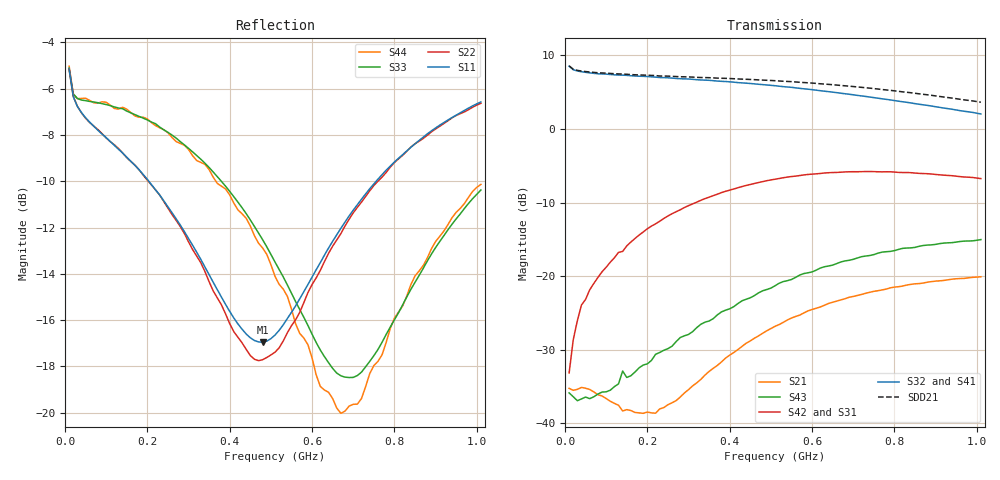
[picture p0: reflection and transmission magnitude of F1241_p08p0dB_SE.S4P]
! Integrated Device Technology
! Corporate Headquarters
! 6024 Silver Creek Valley Road
! San Jose, CA 95138  USA
! Phone:  1-408-284-8200
! Toll Free:  1-800-223-1366
! Webpage:  http://www.idt.com/
! Timing and RF Division
! 515 Groton Road, Suite 102
! Westford, MA 01886-6024
! Device:  F1241
! Description: Dual Intermediate Frequency Digital Variable Gain Amplifier
! Frequency:  10.0 -  500.00 MHz
! Package:  5x5 mm QFN Plastic Package: 32 pin
! Ports:  8 RF, 20 DC
!  Pin  1  = GA3  Pin 17  = RF OUT_B+
!  Pin  2  = GA4  Pin 18  = RF OUT_B-
!  Pin  3  = GA5  Pin 19  = STBY_B
!  Pin  4  = ISET_A  Pin 20  = Ground
!  Pin  5  = ISET_B  Pin 21  = Ground
!  Pin  6  = GB5  Pin 22  = STB_A
!  Pin  7  = GB4  Pin 23  = RF OUT_A-  = Port 4
!  Pin  8  = GB3  Pin 24  = RF OUT_A+  = Port 3
!  Pin  9  = GB2  Pin 25  = NO CONNECT
!  Pin 10  = GB1  Pin 26  = NO CONNECT
!  Pin 11  = RF IN_B+  Pin 27  = VCC
!  Pin 12  = RF IN_B-  Pin 28  = Ground
!  Pin 13  = Ground  Pin 29  = RF IN_A-  = Port 2
!  Pin 14  = VCC  Pin 30  = RF IN_A+  = Port 1
!  Pin 15  = NO CONNECT  Pin 31  = GA1
!  Pin 16  = NO CONNECT  Pin 32  = GA2
!  Pin 16  = GB0  Pin 32  = GA2 / CSb
! State:  12
! Gain State:  8.0 dB
! Voltages:  Vcc = +5.00 Volts  Icc approximately 160.0 mA or 80 mA per channel.
! Data:  The device was measured on a custom evaluation board which has
!  individual transmission lines to the RF pins.  Data was collected
!  using a calibrated network analyzer.  The evaluation board was
!  de-embedded using a port reference technique.
!  The reference plane is the edge of the package pin.
!  Only Channel A was measured.
!  This data is in single-ended operation.  If your needs are balanced
!  or differential S-parameters then this file needs to be used a
!  linear simulator.
! Misc:  Lot Code  160028MY
!  Action Tracker AT004
! Date Measured:  2014-08-14
! Date:  2014-08-28  MJV
! Note:
!  Integrated Device Technology supplies this data as a sample of measured
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# Hz S dB R 50
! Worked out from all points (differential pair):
!   101 points, 10 MHz to 1.01 GHz, reference 50 ohm
!   strongest paths, dB at 10 MHz, 260 MHz, 510 MHz, 760 MHz, 1.01 GHz:
!     S32: 8.5, 6.9, 5.9, 4.2, 2.0
!     S41: 8.6, 6.9, 5.8, 4.1, 1.9
!     S42: -33.2, -11.5, -6.8, -5.8, -6.7
!     S31: -33.1, -11.5, -6.9, -5.9, -6.8
!     S43: -35.9, -29.5, -21.3, -16.9, -15.0
!     S21: -35.2, -37.2, -26.8, -22.0, -20.1
!   taken as a pair (ports 2,1 in; 3,4 out), SDD21 dB: 8.6, 7.2, 6.6, 5.4, 3.6
!   lowest |S11| = -17.0 dB at 480 MHz (marker M1), VSWR 1.33, Z = 39.9 - j7.86 ohm
!   |S11| at or under -10 dB: 203.7 MHz to 755.6 MHz (551.9 MHz wide, 115 % of centre)
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1e7  -5.15 -22.0  -35.26 -9.2  -60.41 64.0  -17.31 14.8
     -35.25 -9.6  -5.17 -21.7  -17.34 14.5  -59.31 65.2
     -33.12 64.3  8.53 177.8  -5.11 -20.5  -36.02 176.5
     8.56 177.9  -33.16 63.4  -35.87 176.6  -5.03 -20.6
5e7  -7.25 -18.7  -35.29 -1.8  -45.83 74.4  -17.35 -1.6
     -35.24 -1.9  -7.28 -18.2  -17.31 -1.7  -45.95 75.4
     -23.06 58.0  7.70 170.0  -6.52 -9.4  -36.66 158.6
     7.71 169.7  -23.16 57.7  -36.43 156.4  -6.41 -9.4
1.4e8  -8.78 -32.0  -38.07 11.6  -37.58 68.9  -17.58 -8.3
       -38.33 8.6  -8.78 -30.6  -17.53 -8.1  -37.58 68.8
       -16.60 52.9  7.31 157.4  -6.87 -16.1  -33.44 145.0
       7.31 156.9  -16.64 52.5  -32.90 142.4  -6.80 -15.3
3.2e8  -13.07 -69.0  -33.44 67.5  -31.21 51.4  -17.26 -17.3
       -34.50 69.0  -13.24 -65.4  -17.24 -17.1  -31.22 50.2
       -9.95 31.2  6.69 132.8  -8.89 -35.1  -27.76 124.7
       6.66 132.2  -9.95 30.7  -27.00 124.8  -9.11 -33.5
4.8e8  -16.95 -137.2  -27.30 69.6  -28.35 36.2  -16.88 -28.4
       -27.77 74.0  -17.71 -136.2  -16.76 -28.3  -28.32 33.9
       -7.19 6.5  6.02 111.2  -12.53 -58.7  -22.82 106.1
       5.95 110.5  -7.15 5.2  -21.99 103.3  -12.88 -55.9
6.7e8  -12.03 152.8  -23.13 54.5  -26.29 19.3  -16.85 -44.2
       -23.23 59.0  -12.26 150.9  -16.61 -44.3  -26.29 15.6
       -5.92 -23.4  4.86 86.7  -18.41 -123.5  -18.79 80.3
       4.75 85.9  -5.88 -25.3  -18.07 78.2  -20.03 -127.8
1.01e9  -6.57 115.3  -20.37 28.0  -24.32 -9.0  -18.09 -70.8
        -20.09 30.3  -6.63 114.5  -17.61 -71.3  -24.39 -13.5
        -6.84 -67.5  2.04 48.8  -10.38 143.2  -15.62 38.9
        1.87 48.2  -6.75 -70.7  -15.04 37.3  -10.13 138.1
